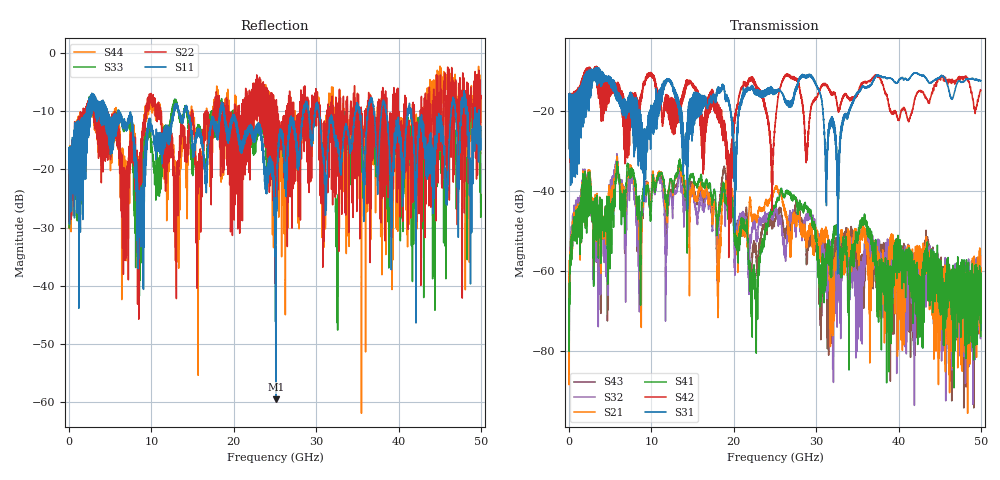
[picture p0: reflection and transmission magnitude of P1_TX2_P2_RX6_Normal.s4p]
!Keysight Technologies,N5225B,MY57041031,A.13.20.10
!Date: Friday, May 31, 2019 11:36:48
!Correction: S11(Full 4 Port(1,2,3,4))
!S12(Full 4 Port(1,2,3,4))
!S13(Full 4 Port(1,2,3,4))
!S14(Full 4 Port(1,2,3,4))
!S21(Full 4 Port(1,2,3,4))
!S22(Full 4 Port(1,2,3,4))
!S23(Full 4 Port(1,2,3,4))
!S24(Full 4 Port(1,2,3,4))
!S31(Full 4 Port(1,2,3,4))
!S32(Full 4 Port(1,2,3,4))
!S33(Full 4 Port(1,2,3,4))
!S34(Full 4 Port(1,2,3,4))
!S41(Full 4 Port(1,2,3,4))
!S42(Full 4 Port(1,2,3,4))
!S43(Full 4 Port(1,2,3,4))
!S44(Full 4 Port(1,2,3,4))
!S4P File: Measurements: <S11,S12,S13,S14>,
!<S21,S22,S23,S24>,
!<S31,S32,S33,S34>,
!<S41,S42,S43,S44>:
# Hz S  dB  R 50.0
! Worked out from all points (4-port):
!   5000 points, 10 MHz to 50 GHz, reference 50 ohm
!   strongest paths, dB at 10 MHz, 12.51 GHz, 25.01 GHz, 37.51 GHz, 50 GHz:
!     S31: -19.5, -13.0, -15.4, -11.1, -12.5
!     S42: -19.5, -17.0, -23.8, -11.5, -15.0
!     S41: -67.0, -38.2, -43.7, -58.9, -76.4
!     S21: -57.5, -38.4, -39.5, -58.2, -61.5
!     S32: -60.4, -43.8, -45.1, -57.8, -66.7
!     S43: -73.2, -41.9, -47.4, -57.2, -67.3
!   lowest |S11| = -59.6 dB at 25.1 GHz (marker M1), VSWR 1.00, Z = 49.9 + j0.0914 ohm
!   |S11| at or under -10 dB: 6.091 GHz to 12.71 GHz (6.616 GHz wide, 70.4 % of centre); 18.82 GHz to 28.43 GHz (9.605 GHz wide, 40.7 % of centre); 41.58 GHz to 46.39 GHz (4.81 GHz wide, 10.9 % of centre)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
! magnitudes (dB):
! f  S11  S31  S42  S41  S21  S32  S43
! 10 MHz  -19.8  -19.5  -19.5  -67.0  -57.5  -60.4  -73.2
! 5.86 GHz  -12.4  -17.5  -14.4  -32.7  -31.7  -31.5  -32.5
! 19.46 GHz  -12.8  -18.6  -32.5  -45.5  -42.3  -41.9  -42.2
! 22.67 GHz  -13.1  -15.0  -13.5  -68.1  -46.7  -49.7  -54.8
! 25.1 GHz  -59.6  -15.1  -21.9  -43.3  -38.9  -44.2  -46.1
! 31.91 GHz  -11.7  -23.3  -16.0  -54.6  -60.1  -61.9  -64.0
! 50 GHz  -12.7  -12.5  -15.0  -76.4  -61.5  -66.7  -67.3
